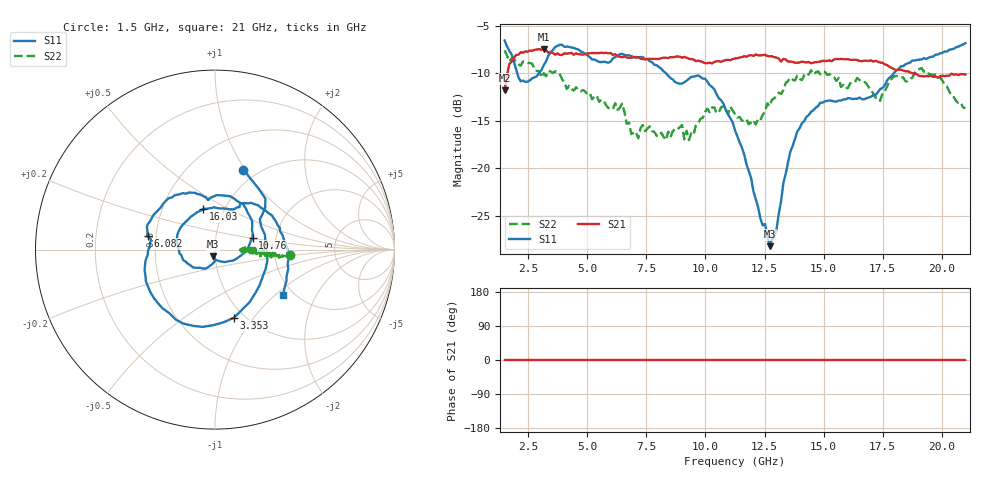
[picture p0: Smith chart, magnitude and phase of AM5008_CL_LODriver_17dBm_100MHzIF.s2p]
!Keysight Technologies,N5245B,MY58422270,A.16.20.02
!Mixer S2P File: Scalar Mixer Measurement
!Calibration State: On
!Parameters: Stimulus Freq, S11, SC21, SC12, S22
# Hz  S  DB  R  50.0
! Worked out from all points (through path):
!   201 points, 1.5 GHz to 21 GHz, reference 50 ohm
!   highest |S21| = -7.41 dB at 3.158 GHz (marker M1); lowest = -11.8 dB at 1.5 GHz (marker M2)
!   lowest |S11| = -28.2 dB at 12.71 GHz (marker M3), VSWR 1.08, Z = 48.9 - j3.68 ohm
!   |S11| at or under -10 dB: 2.039 GHz to 2.946 GHz (907.6 MHz wide, 36.4 % of centre); 8.334 GHz to 17.97 GHz (9.633 GHz wide, 73.3 % of centre)
!   |S22| runs from -17.0 to -7.6 dB; largest |S21 - S12| = 0.43
!   S11 on the Smith chart (normalised r, x): 1.5 GHz: 0.86, +0.98; 3.353 GHz: 0.90, -0.80; 6.082 GHz: 0.45, +0.08; 10.76 GHz: 1.51, +0.21; 16.03 GHz: 0.80, +0.38; 21 GHz: 1.75, -1.13
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1.5e9  -6.53 70.4  -11.79 0.0  -200.00 90.0  -7.57 -4.4
1.7925e9  -7.98 45.3  -8.76 0.0  -200.00 90.0  -8.43 -4.3
2.1825e9  -10.83 26.9  -7.77 0.0  -200.00 90.0  -9.18 -5.5
3.1575e9  -9.12 -56.3  -7.41 0.0  -200.00 90.0  -9.98 -7.6
3.3525e9  -8.10 -74.2  -7.82 0.0  -200.00 90.0  -9.73 -4.1
4.1325e9  -7.16 -131.9  -7.91 0.0  -200.00 90.0  -11.63 -2.8
4.815e9  -7.77 -163.6  -8.02 0.0  -200.00 90.0  -11.75 -6.7
6.0825e9  -8.41 168.5  -8.05 0.0  -200.00 90.0  -13.75 -1.0
8.0325e9  -9.33 111.9  -8.47 0.0  -200.00 90.0  -16.63 -1.5
9.69e9  -10.20 74.0  -8.65 0.0  -200.00 90.0  -15.22 -0.6
1.07625e10  -13.18 17.6  -8.66 0.0  -200.00 90.0  -13.44 -4.1
1.125e10  -15.99 -8.0  -8.42 0.0  -200.00 90.0  -14.26 -3.3
1.21275e10  -23.24 -68.9  -8.00 0.0  -200.00 90.0  -15.39 0.9
1.27125e10  -28.19 -105.2  -8.20 0.0  -200.00 90.0  -13.45 -6.0
1.3005e10  -26.42 -91.7  -8.33 0.0  -200.00 90.0  -12.32 -1.1
1.359e10  -18.26 -118.7  -8.74 0.0  -200.00 90.0  -10.45 -5.2
1.4565e10  -13.88 179.6  -8.85 0.0  -200.00 90.0  -10.09 -6.2
1.60275e10  -12.60 106.5  -8.49 0.0  -200.00 90.0  -11.54 -3.5
1.73925e10  -11.64 62.9  -8.85 0.0  -200.00 90.0  -12.88 -4.1
1.77825e10  -10.45 58.9  -9.30 0.0  -200.00 90.0  -10.77 -4.5
1.91475e10  -8.53 21.3  -10.27 0.0  -200.00 90.0  -9.43 -3.7
2.1e10  -6.81 -34.0  -10.12 0.0  -200.00 90.0  -13.66 -0.6
